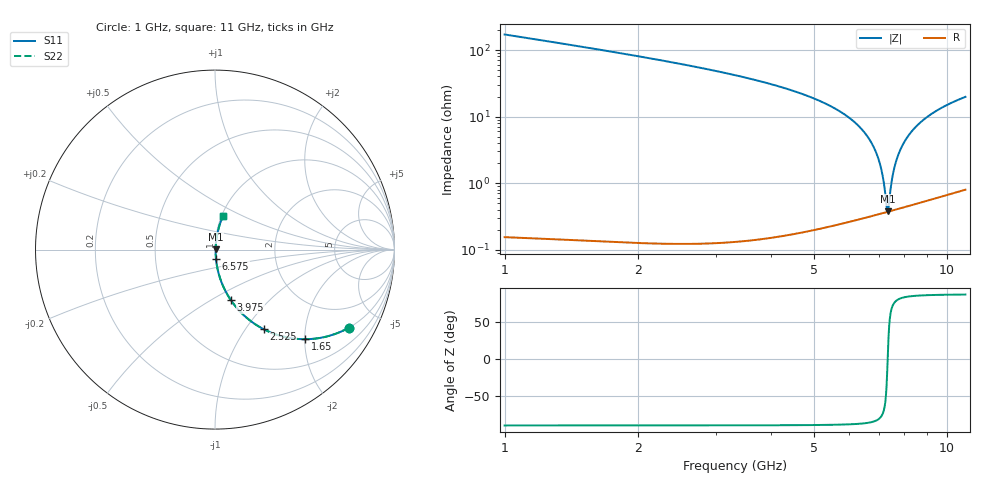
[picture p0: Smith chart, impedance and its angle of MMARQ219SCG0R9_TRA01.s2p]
! MMARQ219SCG0R9_TRA01  S-PARAMETER MODEL  ( General Type )
! Model Generated by TAIYO YUDEN Corporation (http://www.ty-top.com)
! Version 1.0
! TAIYO YUDEN Control No. 160201
! Copyright(c) 2016 TAIYO YUDEN CO.,LTD. All Rights Reserved.
! Product Description (link to TY-COMPAS)
! https://ds.yuden.co.jp/TYCOMPAS/or/detail?pn=MMARQ219SCG0R9BTRA01&u=M
! Products Name : Multilayer Ceramic Capacitors
! Characteristics :
!  Capacitance : 0.9 pF , Rated Voltage : 250V , TCC : CG / C0G
!  Case Size : 2.0 x 1.25 / 0.079 x 0.049 [mm/inch] , Thickness : 0.85 / 0.033 [mm/inch]
!  (Conditions: Temperature = 25 degC , DC Bias Current/Voltage = 0A / 0V)
! External Node Assignments :
!  1  o---| |---o  2
! GND o---------o GND
! Frequency Range : 1000MHz  -  11000MHz  [ 401 STEP ]
# MHz S RI R 50
! Freq[MHz].  S11 Real  S11 Imag  S21 Real  S21 Imag  S12 Real  S12 Imag  S22 Real  S22 Imag
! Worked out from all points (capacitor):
!   401 points, 1 GHz to 11 GHz, reference 50 ohm
!   read as one part in series: C = 912 fF near 1.05 GHz
!   lowest |Z| = 376 mohm at 7.35 GHz (marker M1)
!   series resonance near 7.34 GHz, so ESL is about 520 pH
!   S11 on the Smith chart (normalised r, x): 1 GHz: 1.00, -3.43; 1.65 GHz: 1.00, -2.01; 2.525 GHz: 1.00, -1.22; 3.975 GHz: 1.00, -0.62; 6.575 GHz: 1.01, -0.10; 11 GHz: 1.02, +0.40
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1000  0.7456 -0.4351  0.2544 0.4351  0.2544 0.4351  0.7456 -0.4351
1650  0.5023 -0.4993  0.4977 0.4993  0.4977 0.4993  0.5023 -0.4993
2525  0.2715 -0.4437  0.7285 0.4437  0.7285 0.4437  0.2715 -0.4437
2675  0.2432 -0.428  0.7568 0.428  0.7568 0.428  0.2432 -0.428
3975  0.0891 -0.2825  0.9109 0.2825  0.9109 0.2825  0.0891 -0.2825
4350  0.0649 -0.2432  0.9351 0.2432  0.9351 0.2432  0.0649 -0.2432
5300  0.0263 -0.1533  0.9737 0.1533  0.9737 0.1533  0.0263 -0.1533
6000  0.0118 -0.0952  0.9882 0.0952  0.9882 0.0952  0.0118 -0.0952
6575  0.00575 -0.052  0.9942 0.052  0.9942 0.052  0.00575 -0.052
6825  0.00442 -0.0344  0.9956 0.0344  0.9956 0.0344  0.00442 -0.0344
7025  0.00384 -0.0207  0.9962 0.0207  0.9962 0.0207  0.00384 -0.0207
7175  0.00365 -0.0108  0.9963 0.0108  0.9963 0.0108  0.00365 -0.0108
7300  0.00365 -0.0026  0.9963 0.0026  0.9963 0.0026  0.00365 -0.0026
7350  0.00369 0.000624  0.9963 -0.000624  0.9963 -0.000624  0.00369 0.000624
7400  0.00375 0.00383  0.9962 -0.00383  0.9962 -0.00383  0.00375 0.00383
7525  0.00399 0.0117  0.996 -0.0117  0.996 -0.0117  0.00399 0.0117
7675  0.00444 0.021  0.9956 -0.021  0.9956 -0.021  0.00444 0.021
7925  0.00555 0.0361  0.9944 -0.0361  0.9944 -0.0361  0.00555 0.0361
8275  0.0078 0.0564  0.9922 -0.0564  0.9922 -0.0564  0.0078 0.0564
8750  0.012 0.0825  0.988 -0.0825  0.988 -0.0825  0.012 0.0825
9350  0.0189 0.1133  0.9811 -0.1133  0.9811 -0.1133  0.0189 0.1133
11000  0.0446 0.1872  0.9554 -0.1872  0.9554 -0.1872  0.0446 0.1872
